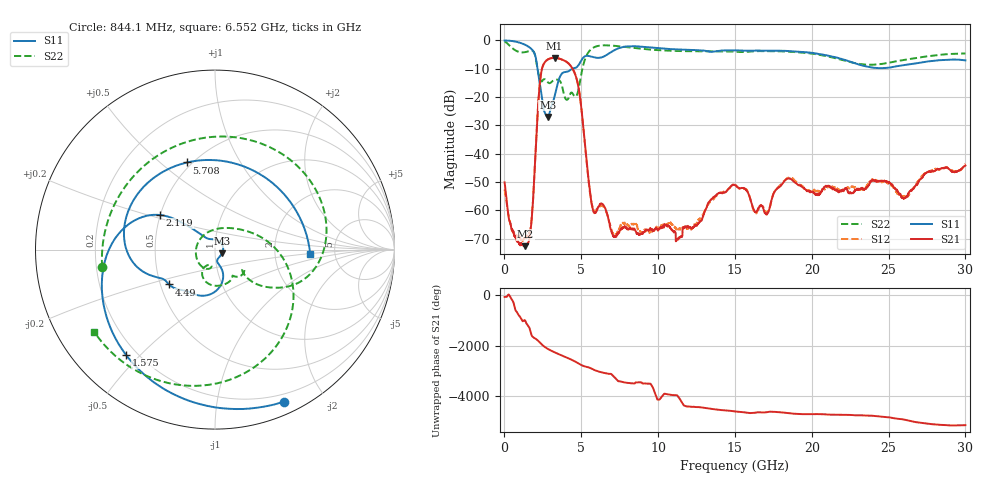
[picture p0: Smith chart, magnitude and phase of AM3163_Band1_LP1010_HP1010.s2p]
!Agilent Technologies,E8364B,MY43040894,A.07.50.67
!Agilent E8364B: A.07.50.67
!Date: Thursday, August 20, 2020 11:21:29
!Correction: S11(Full 2 Port(1,2))
!S21(Full 2 Port(1,2))
!S12(Full 2 Port(1,2))
!S22(Full 2 Port(1,2))
!S2P File: Measurements: S11, S21, S12, S22:
# Hz S  dB  R 50
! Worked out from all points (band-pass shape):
!   3201 points, 10 MHz to 30 GHz, reference 50 ohm
!   highest |S21| = -6.22 dB at 3.262 GHz (marker M1); lowest = -72.6 dB at 1.35 GHz (marker M2)
!   |S21| within 3 dB of the highest: 2.487 GHz to 4.336 GHz (1.849 GHz wide, 54.2 % of centre)
!   lowest |S11| = -27.1 dB at 2.822 GHz (marker M3), VSWR 1.09, Z = 54 - j2.34 ohm
!   |S11| at or under -10 dB: 2.149 GHz to 4.421 GHz (2.272 GHz wide, 69.2 % of centre)
!   |S22| runs from -21.0 to -0.4 dB; largest |S21 - S12| = 0.0054
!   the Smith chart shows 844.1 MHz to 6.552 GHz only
!   S11 on the Smith chart (normalised r, x): 844.1 MHz: 0.12, -1.55; 1.575 GHz: 0.16, -0.45; 2.119 GHz: 0.50, +0.22; 4.49 GHz: 0.56, -0.24; 5.708 GHz: 0.47, +0.62; 6.552 GHz: 3.25, -0.21
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1e7  -0.07 -5.1  -50.11 -58.4  -52.63 110.9  -0.44 -17.2
3.942469e8  -0.20 -30.2  -64.80 -80.9  -64.78 -46.2  -2.22 -90.7
8.440969e8  -0.63 -65.6  -71.11 21.5  -69.05 -117.1  -3.93 -171.2
1.350178e9  -1.60 -108.4  -72.61 75.0  -69.92 176.2  -4.18 109.9
1.575103e9  -2.29 -130.2  -70.98 -155.0  -68.87 -72.6  -3.88 73.4
2.118672e9  -8.80 147.9  -29.49 35.3  -29.43 35.3  -9.16 -36.5
2.821562e9  -27.05 -29.1  -6.77 31.7  -6.78 31.7  -14.81 -54.6
3.262041e9  -19.84 -72.2  -6.22 -105.1  -6.23 -105.1  -14.03 -70.9
3.852469e9  -11.33 -110.0  -7.06 99.1  -7.06 99.2  -18.66 -121.2
4.489756e9  -9.87 -142.8  -10.61 -77.8  -10.59 -77.7  -19.25 -167.7
5.014581e9  -6.97 -168.1  -24.41 104.0  -24.37 103.8  -11.57 15.5
5.7081e9  -5.85 107.8  -58.55 -45.8  -58.21 -43.4  -2.88 -79.8
6.551569e9  -5.50 -2.5  -59.13 146.7  -59.51 141.5  -1.78 -145.8
7.35755e9  -2.97 -95.0  -68.17 -151.3  -67.64 -37.2  -2.07 170.5
8.275994e9  -2.10 -168.4  -66.44 97.9  -64.71 105.2  -2.63 129.5
1.000979e10  -2.80 99.9  -66.93 168.3  -66.25 73.8  -3.50 62.1
1.223092e10  -3.44 10.8  -66.13 -118.9  -66.03 -109.6  -3.87 -14.5
1.5005e10  -3.56 -71.5  -51.12 58.0  -51.01 60.6  -4.03 -93.3
2.000958e10  -4.44 163.4  -53.53 -47.7  -53.21 -51.3  -4.70 136.6
2.275554e10  -8.03 60.4  -53.51 -90.9  -51.81 -92.6  -8.01 21.3
2.500479e10  -9.66 -62.3  -50.20 -174.5  -50.06 -175.5  -7.98 -92.3
3e10  -7.10 105.0  -44.20 -128.7  -43.53 -133.3  -4.64 102.7
